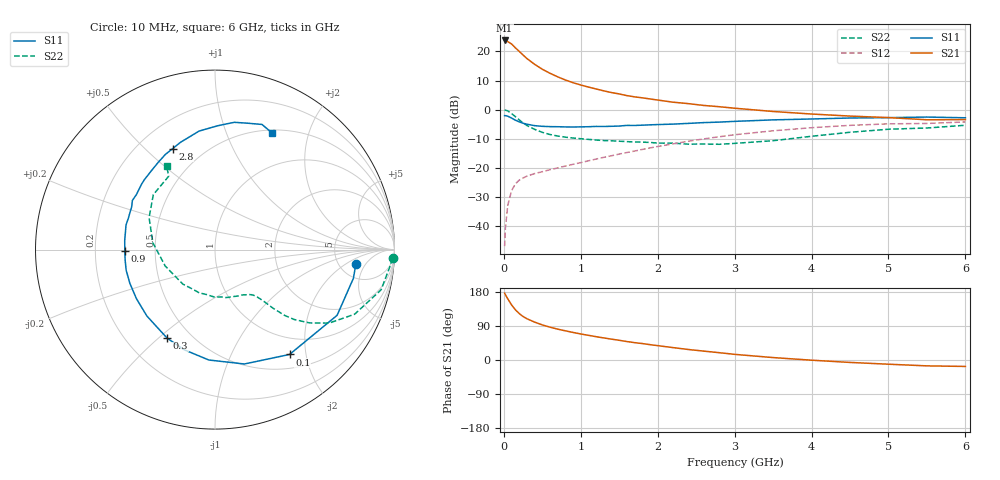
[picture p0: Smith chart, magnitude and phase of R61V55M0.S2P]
! SIEMENS Small Signal Semiconductors
! BFR193
! Si NPN RF Bipolar Junction Transistor in SOT23
! VCE = 1.5 V  IC = 5 mA
! Common Emitter S-Parameters:  May  1996
# GHz  S  MA  R  50
!  f  S11  S21  S12  S22
! GHz  MAG  ANG  MAG  ANG  MAG  ANG  MAG  ANG
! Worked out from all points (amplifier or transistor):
!   36 points, 10 MHz to 6 GHz, reference 50 ohm
!   highest |S21| = 23.8 dB at 10 MHz (marker M1)
!   |S21| within 3 dB of that: start of sweep to 169 MHz
!   unconditionally stable (mu >= 1): 882.8 MHz to 2.083 GHz
!   at 250 MHz: K = 0.43, MSG = 21.1 dB, |S12| = -23.5 dB
!   at 1.4 GHz: K = 1.07, MAG = 9.2 dB, |S12| = -15.9 dB
!   at 6 GHz: K = 0.98, MSG = 0.4 dB, |S12| = -4.2 dB
!   S11 on the Smith chart (normalised r, x): 10 MHz: 7.09, -3.09; 100 MHz: 0.71, -1.71; 300 MHz: 0.37, -0.53; 900 MHz: 0.33, -0.00; 2.8 GHz: 0.34, +0.61; 6 GHz: 0.53, +1.46
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0.01  0.7886 -6.0  15.44 176.5  0.0045 85.1  0.9903 -2.8
0.02  0.7877 -11.7  15.24 172.4  0.0091 85.4  0.9788 -5.6
0.05  0.7725 -28.3  14.78 161.7  0.0223 75.9  0.9523 -13.6
0.1  0.7168 -54.6  13.44 145.6  0.0404 65.1  0.8576 -24.8
0.15  0.658 -75.6  11.52 132.5  0.0529 56.9  0.7562 -32.8
0.2  0.6161 -93.2  10.03 122.6  0.0614 51.7  0.6664 -37.8
0.25  0.5837 -107.2  8.671 114.7  0.0668 48.2  0.5892 -41.4
0.3  0.5608 -118.4  7.55 108.9  0.0719 46.6  0.5332 -43.4
0.4  0.53 -135.8  6.008 100.0  0.0795 45.5  0.4583 -45.3
0.5  0.5161 -148.0  4.937 92.6  0.0857 46.3  0.4065 -46.4
0.6  0.5102 -158.5  4.213 86.6  0.0927 47.5  0.3735 -47.4
0.7  0.5081 -166.9  3.661 81.4  0.0995 49.0  0.352 -48.4
0.9  0.5024 -179.4  2.9 72.7  0.1149 51.6  0.3247 -50.8
1.1  0.5079 169.6  2.44 65.1  0.1319 54.4  0.3079 -54.9
1.3  0.5133 160.2  2.099 58.2  0.1514 56.0  0.2941 -59.3
1.6  0.5357 149.2  1.74 48.7  0.1833 56.8  0.2817 -68.1
2.2  0.5634 129.4  1.342 32.7  0.2581 54.6  0.2649 -90.4
2.8  0.6102 112.7  1.122 19.3  0.3418 47.9  0.2536 -121.7
3.5  0.6664 97.6  0.929 6.4  0.4327 37.0  0.2922 -161.8
4.5  0.7173 81.4  0.774 -6.4  0.5364 20.3  0.408 154.2
5.5  0.7448 69.4  0.669 -15.5  0.5781 3.8  0.4832 122.3
6  0.724 64.1  0.674 -17.0  0.6139 -1.1  0.5384 120.0
